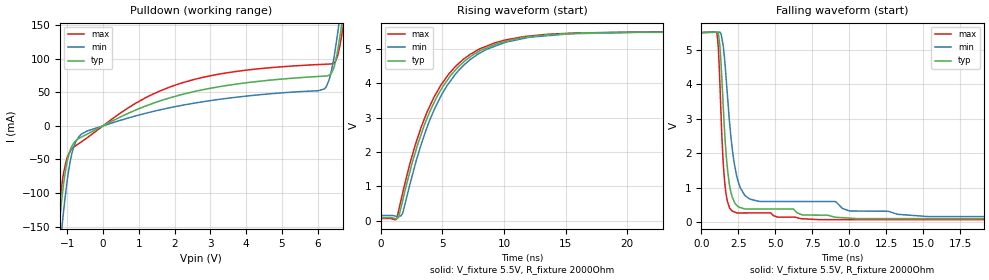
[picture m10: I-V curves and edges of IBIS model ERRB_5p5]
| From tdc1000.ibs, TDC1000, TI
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|   Model
[Model]   ERRB_5p5
Model_type   Open_drain
Polarity   Non-Inverting
Vmeas = 2.25
Vref = 5.5
Cref = 1pF
Rref = 2000
|   typ   min   max
C_comp   0.791pF   0.756pF   0.854pF
[Voltage Range]   5.5   5.499   5.501
[Temperature Range]   27   125   -40
[Pullup Reference]   5.5   5.499   5.501
[Pulldown Reference]   0   0   0
[Power Clamp Reference]   5.5   5.499   5.501
[GND Clamp Reference]   0   0   0
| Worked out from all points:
|   slope of the pulldown table from 0 to 0.825 V, typ, clamps not added: 38.5 ohm
|   falling waveform, V_fixture 5.5V, R_fixture 2000Ohm: 20-80 % time 514ps typ, 826ps min, 362ps max; typ from 5.5 V to 0.096 V
|   rising waveform, V_fixture 5.5V, R_fixture 2000Ohm: 20-80 % time 3.94ns typ, 3.97ns min, 3.85ns max; typ from 0.096 V to 5.5 V
[Pulldown]
|   Voltage   I(typ)   I(min)   I(max)
-5.5V     -2.944A    -2.976A    -2.92A
-1.375V   -232.9mA   -279.5mA   -206mA
-1.226V   -146.7mA   -192.4mA   -121.5mA
-1.144V   -104.1mA   -147.5mA   -84.12mA
-896.5mV  -33.28mA   -46.78mA   -35.99mA
-599.5mV  -16.48mA   -12.07mA   -23.6mA
2.139V    45.61mA    29.77mA    62.62mA
6.182V    73.84mA    54.56mA    91.43mA
6.446V    84.77mA    97.54mA    92.68mA
6.628V    133mA      163.6mA    119.5mA
6.726V    170.9mA    206.2mA    151.2mA
11V       2.462A     2.537A     2.388A
[Ramp]
R_load = 2000
|   typ   min   max
dV/dt_r   3.24226/3.94022e-09   3.2066/3.96748e-09   3.2607/3.84733e-09
dV/dt_f   3.24226/5.13413e-10   3.2066/8.26466e-10   3.2607/3.61772e-10
[Falling Waveform]
V_fixture = 5.5V
V_fixture_min = 5.499V
V_fixture_max = 5.501V
R_fixture = 2000Ohm
C_fixture = 0F
|   Time   V(typ)   V(min)   V(max)
0s        5.5V       5.499V     5.501V
1.024ns   5.514V     5.51V      5.518V
1.156ns   5.462V     5.512V     4.977V
1.402ns   4.034V     5.302V     2.358V
1.626ns   2.265V     4.455V     965.2mV
1.961ns   940.6mV    2.641V     378.2mV
2.402ns   481.7mV    1.315V     264.6mV
3.842ns   377.4mV    602.5mV    263.7mV
15.34ns   96.9mV     156.4mV    66.8mV
100ns     96.24mV    154.7mV    66.5mV
[Rising Waveform]
V_fixture = 5.5V
V_fixture_min = 5.499V
V_fixture_max = 5.501V
R_fixture = 2000Ohm
C_fixture = 0F
|   Time   V(typ)   V(min)   V(max)
0s        96.24mV    154.7mV    66.5mV
1.237ns   58.89mV    132.7mV    36.84mV
1.454ns   108.7mV    117.7mV    296.7mV
1.755ns   555mV      204mV      774mV
3.349ns   2.597V     2.303V     2.796V
4.367ns   3.474V     3.262V     3.63V
5.501ns   4.146V     3.997V     4.266V
7.891ns   4.92V      4.855V     4.981V
11.69ns   5.346V     5.319V     5.37V
100ns     5.5V       5.499V     5.501V
